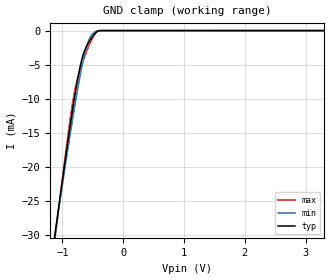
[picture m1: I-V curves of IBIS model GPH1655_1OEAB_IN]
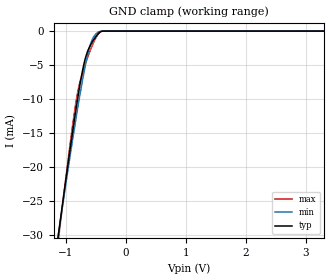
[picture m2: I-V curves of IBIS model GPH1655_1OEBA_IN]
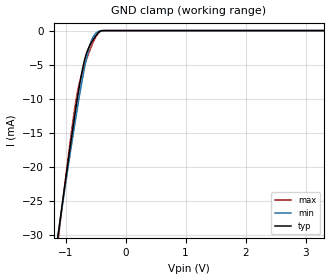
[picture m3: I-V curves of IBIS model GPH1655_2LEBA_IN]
| TEXAS INSTRUMENTS INCORPORATED
| Standard Linear and Logic Group
| IBIS Model of SN74GTLPH1655
| 16-Bit LVTTL-to-GTLP Adjustable-Edge-Rate Universal Bus Transceiver
| This file contains package information for the following:
|  TSSOP 64-pin (DGG) package as [Component] GTLPH1655_DGG
| This device can be powered at the following Vccs:
|  3.3 volt Vcc
| This file provides unique models under the [Model Selector] for each Vcc.
| For operation at a specific Vcc, select the appropriate model after each
| [Model Selector] keyword.
[IBIS Ver]   3.2
[Comment char]  |_char
[File Name]   sn74gtlph1655.ibs
[File Rev]   1.2 | b_die
[Date]   February 19, 2004
[Source]   Data created from TI-SPICE simulations at TI-SLL.
[Notes]   The following is an IBIS list for the GTLPH1655.
   Please contact sllibis@ti.com with questions and
   comments concerning SLL IBIS models.
   - FILE REV HISTORY
   - 1.2 Release New IBIS file on 02/26/04
   - Power-clamp data has been deleted since there is no
   power-clamp diode in the device.
   - In the B-port output model, we varied across process,
   temperature, and voltage, but VTT is constant.
   - Non-monotonic data in ground-clamp due to bus-hold.
[Disclaimer] Property of Texas Instruments Incorporated.  Unauthorized
   reproduction and/or distribution is strictly prohibited.
   This product is protected under copyright law.
   Created  2002, (C) Copyright  2002, Texas Instruments
   Incorporated, All Rights Reserved
   UNLESS THERE IS A SIGNED, WRITTEN AGREEMENT TO THE
   CONTRARY, TEXAS INSTRUMENTS (TI) IS PROVIDING THE IBIS
   MODELS  AND WITHOUT ANY WARRANTY, EXPRESSED OR
   IMPLIED.  TI assumes no liability for:
   1) the accuracy of the IBIS models provided to your
   company;
   2) the proper functioning of these IBIS Models in your
   design or for any resulting applications; or
   3) infringement of patents, copyrights or intellectual
   property rights resulting from your use of these IBIS
   models.
   TI provides IBIS Models as a service to our customers.
   You and your company shall not distribute, sell or give
   these models to anyone else without prior written
   permission from TI.
   TI reserves the right to make changes to our products or
   to discontinue any semiconductor product or service
   without notice, and advises our customers to obtain the
   latest version of relevant information to verify, before
   placing orders, that the information being relied on is
   current.
   Please be aware that your receipt and use of the IBIS
   information provided shall serve as acceptance of these
   terms and conditions.  If you do not accept these terms,
   you should return or destroy the IBIS models and any
   other accompanying information immediately.
| Component GTLPH1655_DGG 64-pin TSSOP
[Component]   GTLPH1655_DGG
[Manufacturer]   Texas Instruments, Inc.
[Package]
|   typ   min   max
R_pkg   5.500e-02   4.300e-02   7.000e-02
L_pkg   3.686e-09   2.988e-09   4.882e-09
C_pkg   6.250e-13   4.220e-13   9.610e-13
[Pin]   signal_name   model_name   R_pin   L_pin   C_pin
1   N1OEAB   GPH1655_1OEAB_IN   4.600e-02   4.878e-09   9.030e-13
2   N1OEBA   GPH1655_1OEBA_IN   4.600e-02   4.546e-09   9.490e-13
3   VCC   POWER   5.200e-02   4.386e-09   8.450e-13
4   1A1   GPH1655_A_IO   5.800e-02   4.228e-09   7.710e-13
5   GND   GND   6.900e-02   4.189e-09   7.760e-13
6   1A2   GPH1655_A_IO   7.000e-02   3.980e-09   7.760e-13
7   1A3   GPH1655_A_IO   4.900e-02   3.682e-09   6.630e-13
8   GND   GND   5.300e-02   3.630e-09   6.040e-13
9   1A4   GPH1655_A_IO   5.400e-02   3.442e-09   5.440e-13
10   GND   GND   5.300e-02   3.324e-09   5.110e-13
11   1A5   GPH1655_A_IO   5.600e-02   3.297e-09   4.910e-13
12   GND   GND   5.700e-02   3.220e-09   4.640e-13
13   1A6   GPH1655_A_IO   5.700e-02   3.154e-09   4.400e-13
14   1A7   GPH1655_A_IO   5.700e-02   3.096e-09   4.300e-13
15   VCC   POWER   6.000e-02   3.141e-09   4.380e-13
16   1A8   GPH1655_A_IO   5.900e-02   3.057e-09   4.270e-13
17   2A1   GPH1655_A_IO   5.700e-02   2.999e-09   4.230e-13
18   GND   GND   5.900e-02   3.146e-09   4.400e-13
19   2A2   GPH1655_A_IO   5.800e-02   3.109e-09   4.330e-13
20   2A3   GPH1655_A_IO   5.700e-02   3.142e-09   4.410e-13
21   GND   GND   5.700e-02   3.219e-09   4.690e-13
22   2A4   GPH1655_A_IO   5.500e-02   3.259e-09   4.940e-13
23   2A5   GPH1655_A_IO   5.500e-02   3.339e-09   5.190e-13
24   GND   GND   5.400e-02   3.436e-09   5.490e-13
25   2A6   GPH1655_A_IO   5.100e-02   3.492e-09   5.970e-13
26   GND   GND   5.000e-02   3.668e-09   6.700e-13
27   2A7   GPH1655_A_IO   6.700e-02   3.936e-09   7.900e-13
28   VCC   POWER   6.500e-02   4.111e-09   7.920e-13
29   2A8   GPH1655_A_IO   6.000e-02   4.258e-09   7.810e-13
30   GND   GND   5.300e-02   4.392e-09   8.520e-13
31   N2OEAB   GPH1655_2OEAB_IN   4.700e-02   4.598e-09   9.610e-13
32   N2OEBA   GPH1655_2OEBA_IN   4.600e-02   4.882e-09   9.100e-13
33   NOE   GPH1655_NOE_IN   4.400e-02   4.855e-09   9.000e-13
34   2LEBA   GPH1655_2LEBA_IN   4.500e-02   4.542e-09   9.420e-13
35   2LEAB   GPH1655_2LEAB_IN   5.100e-02   4.367e-09   8.360e-13
36   BIASVCC   GPH1655_BIAS_IN   5.900e-02   4.230e-09   7.640e-13
37   2B8   GPH1655_B_IO   6.700e-02   4.155e-09   7.630e-13
38   2B7   GPH1655_B_IO   6.900e-02   3.958e-09   7.660e-13
39   GND   GND   5.000e-02   3.719e-09   6.670e-13
40   2B6   GPH1655_B_IO   4.900e-02   3.493e-09   5.910e-13
41   VREF   GPH1655_VREF_IN   5.200e-02   3.414e-09   5.470e-13
42   2B5   GPH1655_B_IO   5.400e-02   3.326e-09   5.180e-13
43   2B4   GPH1655_B_IO   5.400e-02   3.249e-09   4.890e-13
44   GND   GND   5.600e-02   3.182e-09   4.630e-13
45   2B3   GPH1655_B_IO   5.600e-02   3.112e-09   4.390e-13
46   2B2   GPH1655_B_IO   5.500e-02   3.036e-09   4.260e-13
47   GND   GND   5.500e-02   3.045e-09   4.320e-13
48   2B1   GPH1655_B_IO   5.800e-02   3.010e-09   4.250e-13
49   1B8   GPH1655_B_IO   5.700e-02   2.988e-09   4.220e-13
50   VCC   POWER   5.900e-02   3.126e-09   4.360e-13
51   1B7   GPH1655_B_IO   5.800e-02   3.116e-09   4.300e-13
52   1B6   GPH1655_B_IO   5.600e-02   3.109e-09   4.350e-13
53   GND   GND   5.500e-02   3.176e-09   4.550e-13
54   1B5   GPH1655_B_IO   5.400e-02   3.272e-09   4.810e-13
55   1B4   GPH1655_B_IO   5.300e-02   3.333e-09   5.050e-13
56   1B3   GPH1655_B_IO   5.100e-02   3.378e-09   5.290e-13
57   GND   GND   5.200e-02   3.580e-09   5.820e-13
58   1B2   GPH1655_B_IO   4.800e-02   3.650e-09   6.450e-13
59   1B1   GPH1655_B_IO   6.700e-02   3.899e-09   7.670e-13
60   GND   GND   6.900e-02   4.190e-09   7.660e-13
61   VERC   GPH1655_ERC_IN   6.000e-02   4.270e-09   7.620e-13
62   1LEBA   GPH1655_1LEBA_IN   5.300e-02   4.426e-09   8.350e-13
63   1LEAB   GPH1655_1LEAB_IN   4.800e-02   4.611e-09   9.390e-13
64   CLK   GPH1655_CLK_IN   4.300e-02   4.845e-09   8.930e-13
| Models and submodels in the file (15): GPH1655_1OEAB_IN (Input), GPH1655_1OEBA_IN (Input), GPH1655_2LEBA_IN (Input), GPH1655_2LEAB_IN (Input), GPH1655_ERC_IN (Input), GPH1655_NOE_IN (Input), GPH1655_2OEAB_IN (Input), GPH1655_BIAS_IN (Input), GPH1655_2OEBA_IN (Input), GPH1655_VREF_IN (Input), GPH1655_1LEAB_IN (Input), GPH1655_CLK_IN (Input), GPH1655_1LEBA_IN (Input), GPH1655_A_IO (I/O), GPH1655_B_IO (I/O_open_drain)
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| NOTE:  The [Diff Pin] section is commented out because the ibischk3 program
|   currently flags it as an Error when it shouldn't
| [Diff Pin]  inv_pin   vdiff   tdelay_typ
|37   41   100mv   NA
|38   41   100mv   NA
|40   41   100mv   NA
|42   41   100mv   NA
|43   41   100mv   NA
|45   41   100mv   NA
|46   41   100mv   NA
|48   41   100mv   NA
|49   41   100mv   NA
|51   41   100mv   NA
|52   41   100mv   NA
|54   41   100mv   NA
|55   41   100mv   NA
|56   41   100mv   NA
|58   41   100mv   NA
|59   41   100mv   NA
[Model]   GPH1655_1OEAB_IN
Model_type  Input
Vinl=0.69
Vinh=1.05
| variable   typ   min   max
C_comp   3.07pF   2.22pF   3.87pF
[Temperature Range]   40   100   -40
| Ambient temperature   25   85   -40
[Voltage range]   3.3   3.15   3.45
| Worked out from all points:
|   GND clamp passes 1 mA (typ) near -0.52 V on its own axis
[GND Clamp]
| GPH1655_1OEAB_IN
|   Voltage   I(typ)   I(min)   I(max)
-5.5V     -348mA     -320.7mA   -389.8mA
-1.11V    -29.09mA   -29.13mA   -29.74mA
-1.07V    -26.47mA   -26.72mA   -26.78mA
-895mV    -15.37mA   -16.48mA   -14.42mA
-840mV    -12.09mA   -13.41mA   -10.99mA
-800mV    -9.813mA   -11.24mA   -8.913mA
-725mV    -5.999mA   -7.402mA   -6.269mA
-660mV    -3.579mA   -4.448mA   -4.491mA
-575mV    -1.843mA   -1.603mA   -2.457mA
-485mV    -638.7uA   -307.2uA   -791.6uA
-390mV    -8.587uA   -16.56uA   -7.146uA
3.3V      166.6pA    582.8pA    1.325nA
[Model]   GPH1655_1OEBA_IN
Model_type  Input
Vinl=0.8
Vinh=2.0
| variable   typ   min   max
C_comp   3.07pF   2.23pF   3.90pF
[Temperature Range]   40   100   -40
| Ambient temperature   25   85   -40
[Voltage range]   3.3   3.15   3.45
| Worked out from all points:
|   GND clamp passes 1 mA (typ) near -0.52 V on its own axis
[GND Clamp]
| GPH1655_1OEBA_IN
|   Voltage   I(typ)   I(min)   I(max)
-5.5V     -348mA     -320.7mA   -389.8mA
-1.11V    -29.09mA   -29.13mA   -29.74mA
-1.07V    -26.47mA   -26.72mA   -26.78mA
-895mV    -15.37mA   -16.48mA   -14.42mA
-840mV    -12.09mA   -13.41mA   -10.99mA
-800mV    -9.813mA   -11.24mA   -8.913mA
-725mV    -5.999mA   -7.402mA   -6.269mA
-660mV    -3.579mA   -4.448mA   -4.491mA
-575mV    -1.843mA   -1.603mA   -2.457mA
-485mV    -638.7uA   -307.2uA   -791.6uA
-390mV    -8.587uA   -16.56uA   -7.146uA
3.3V      166.6pA    582.8pA    1.325nA
[Model]   GPH1655_2LEBA_IN
Model_type  Input
Vinl=0.8
Vinh=2.0
| variable   typ   min   max
C_comp   3.01pF   2.26pF   3.95pF
[Temperature Range]   40   100   -40
| Ambient temperature   25   85   -40
[Voltage range]   3.3   3.15   3.45
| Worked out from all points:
|   GND clamp passes 1 mA (typ) near -0.52 V on its own axis
[GND Clamp]
| GPH1655_2LEBA_IN
|   Voltage   I(typ)   I(min)   I(max)
-5.5V     -348mA     -320.7mA   -389.8mA
-1.11V    -29.09mA   -29.13mA   -29.74mA
-1.07V    -26.47mA   -26.72mA   -26.78mA
-895mV    -15.37mA   -16.48mA   -14.42mA
-840mV    -12.09mA   -13.41mA   -10.99mA
-800mV    -9.813mA   -11.24mA   -8.913mA
-725mV    -5.999mA   -7.402mA   -6.269mA
-660mV    -3.579mA   -4.448mA   -4.491mA
-575mV    -1.843mA   -1.603mA   -2.457mA
-485mV    -638.7uA   -307.2uA   -791.6uA
-390mV    -8.587uA   -16.56uA   -7.146uA
3.3V      166.6pA    582.8pA    1.325nA
